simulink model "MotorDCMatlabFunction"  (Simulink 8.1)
settings: Solver=ode45  StartTime=0.0  StopTime=tmax  MaxStep=1e-4  RelTol=1e-3
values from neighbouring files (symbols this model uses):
  Bm = 2.01e-6    (= 2.01e-06)    [MotorDCParam.m]
  Jm = 1.4e-6    (= 1.4e-06)    [MotorDCParam.m]
  K1 = 1/(2*pi)    (= 0.159154943092)    [MotorDCParam.m]
  K2 = 1/25    (= 0.04)    [MotorDCParam.m]
  K3 = 10    [MotorDCParam.m]
  kb = 2.2e-2    (= 0.022)    [MotorDCParam.m]
  Kd1 = K2    (= 0.04)    [MotorDCParam.m]
  Kd2 = 1/1000    (= 0.001)    [MotorDCParam.m]
  Kd3 = 1/1000    (= 0.001)    [MotorDCParam.m]
  Lm = 5.8e-4    (= 0.00058)    [MotorDCParam.m]
  Rm = 5.3    [MotorDCParam.m]
  U = 5    [MotorDCParam.m]

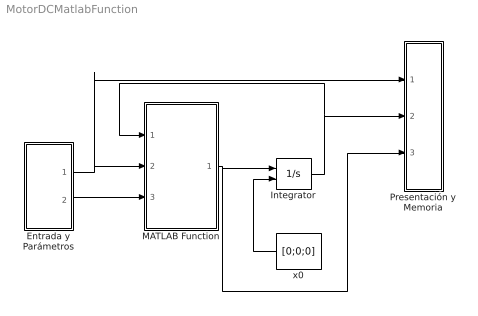
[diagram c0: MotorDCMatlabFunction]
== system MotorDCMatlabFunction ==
  Entrada y Parámetros : Subsystem
  Integrator : Integrator  InitialConditionSource=external  InitialCondition=[0;0]
  MATLAB Function : MATLAB Function  TreatAsAtomicUnit=on
  Presentación y Memoria : Subsystem
  x0 : Constant  Value=[0;0;0]
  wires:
  MATLAB Function/1(dx) -> Presentación y Memoria/3(dx), Integrator/1
  Integrator/1 -> MATLAB Function/1(x), Presentación y Memoria/2(x)
  x0/1 -> Integrator/2
  Entrada y Parámetros/1(um) -> Presentación y Memoria/1(um), MATLAB Function/2(um)
  Entrada y Parámetros/2(params) -> MATLAB Function/3(params)

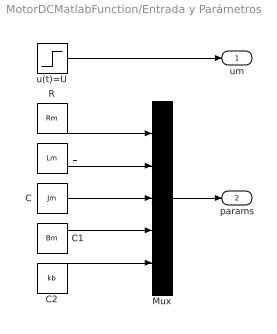
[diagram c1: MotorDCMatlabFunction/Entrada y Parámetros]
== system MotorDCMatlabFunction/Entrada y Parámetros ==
  C : Constant  Value=Jm
  C1 : Constant  Value=Bm
  C2 : Constant  Value=kb
  L : Constant  Value=Lm
  Mux : Mux  Inputs=5
  R : Constant  Value=Rm
  u(t)=U : Step  Time=0  After=U  SampleTime=0
  um : Outport
  params : Outport  Port=2
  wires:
  u(t)=U/1 -> um/1
  R/1 -> Mux/1
  L/1 -> Mux/2
  C/1 -> Mux/3
  Mux/1 -> params/1
  C1/1 -> Mux/4
  C2/1 -> Mux/5

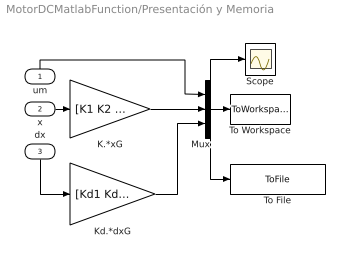
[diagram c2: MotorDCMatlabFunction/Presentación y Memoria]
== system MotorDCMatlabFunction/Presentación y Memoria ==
  um : Inport
  x : Inport  Port=2
  dx : Inport  Port=3
  K.*xG : Gain  Gain=[K1 K2 K3]
  Kd.*dxG : Gain  Gain=[Kd1 Kd2 Kd3]
  Mux : Mux  Inputs=3
  Scope : Scope
  To File : ToFile  Filename=MotFunction.mat  SaveFormat=Timeseries
  To Workspace : ToWorkspace  VariableName=MotEstados  SampleTime=-1
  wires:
  x/1 -> K.*xG/1
  um/1 -> Mux/1
  K.*xG/1 -> Mux/2
  Mux/1 -> To File/1, Scope/1, To Workspace/1
  Kd.*dxG/1 -> Mux/3
  dx/1 -> Kd.*dxG/1

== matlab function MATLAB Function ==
function dx  = MotDCState(x,um,params)
%#codegen
% x1=theta(t); x2=w(t); x3=i(t)
Rm=params(1);
Lm=params(2);
Bm=params(3);
Jm=params(4);
kb=params(5);
km=kb;
A=[0 1 0;0 -Bm/Jm km/Jm;0 -kb/Lm -Rm/Lm];
B=[0;0; 1/Lm];
dx = A*x +B*um;
end
